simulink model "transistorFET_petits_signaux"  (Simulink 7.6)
settings: Solver=ode15s  StartTime=0.0  StopTime=0.06  RelTol=1e-3
InitFcn:
  | clc
  | RD=1000;
libraries: fl_lib x7, nesl_utility x3, AppliElectrical_lib x1

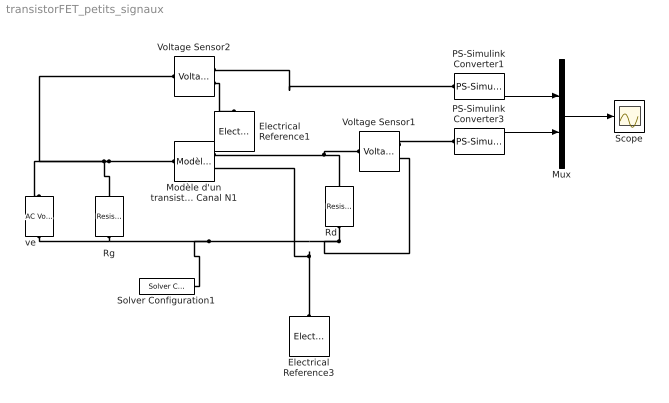
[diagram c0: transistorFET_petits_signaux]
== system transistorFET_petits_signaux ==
  Electrical Reference1 : fl_lib/Electrical/Electrical Elements/Electrical Reference  DialogController=NetworkEngine.DynNeDlgSource  SystemSampleTime=-1  i_Log=off  LocalVarNames=|i  LocalVarDescs=|i  LocalVarLogging=0
  Electrical Reference3 : fl_lib/Electrical/Electrical Elements/Electrical Reference  DialogController=NetworkEngine.DynNeDlgSource  SystemSampleTime=-1  i_Log=off  LocalVarNames=|i  LocalVarDescs=|i  LocalVarLogging=0
  Modèle d'un transistor à effet de champ Canal N1 : AppliElectrical_lib/Modèle d'un transistor à effet de champ Canal N  DialogController=NetworkEngine.DynNeDlgSource  SystemSampleTime=-1  g=0.003 A/V  rho=1e+6 Ohm  ie_Log=off  vgs_Log=off  is_Log=off  vds_Log=off  LocalVarNames=|ie|vgs|is|vds  LocalVarDescs=|courant d'entrée du FET|tension, Grille-Source|courant Drain-Source|tension Drain-Source  LocalVarLogging=[0 0 0 0]
  Mux : Mux  Inputs=2
  PS-Simulink Converter1 : nesl_utility/PS-Simulink Converter  DialogController=NetworkEngine.DynNeUtilDlgSource  SystemSampleTime=-1  PhysicalDomain=network_engine_domain  LeftPortType=input  RightPortType=output  SubClassName=ps_output  Unit=1  AffineConversion=off
  PS-Simulink Converter3 : nesl_utility/PS-Simulink Converter  DialogController=NetworkEngine.DynNeUtilDlgSource  SystemSampleTime=-1  PhysicalDomain=network_engine_domain  LeftPortType=input  RightPortType=output  SubClassName=ps_output  Unit=1  AffineConversion=off
  Rd : fl_lib/Electrical/Electrical Elements/Resistor  DialogController=NetworkEngine.DynNeDlgSource  SystemSampleTime=-1  R=1 kOhm  i_Log=off  v_Log=off  LocalVarNames=|i|v  LocalVarDescs=|i|v  LocalVarLogging=[0 0]
  Rg : fl_lib/Electrical/Electrical Elements/Resistor  DialogController=NetworkEngine.DynNeDlgSource  SystemSampleTime=-1  R=1 MOhm  i_Log=off  v_Log=off  LocalVarNames=|i|v  LocalVarDescs=|i|v  LocalVarLogging=[0 0]
  Scope : Scope
  Solver Configuration1 : nesl_utility/Solver Configuration  DialogController=NetworkEngine.DynNeUtilDlgSource  SystemSampleTime=-1  PhysicalDomain=network_engine_domain  LeftPortType=input  RightPortType=generic  SubClassName=solver  Accelerate=off  Profile=off  ResidualTolerance=1e-9  MaxNonlinIter=3  MaxModeIter=2  DoFixedCost=off  UseLocalSampling=off  DoDC=off  LinearAlgebra=Sparse  LocalSolverSampleTime=.001  LocalSolverChoice=NE_BACKWARD_EULER_ADVANCER  UseLocalSolver=off
  Voltage Sensor1 : fl_lib/Electrical/Electrical Sensors/Voltage Sensor  DialogController=NetworkEngine.DynNeDlgSource  SystemSampleTime=-1  i1_Log=off  v1_Log=off  LocalVarNames=|i1|v1  LocalVarDescs=|i1|v1  LocalVarLogging=[0 0]
  Voltage Sensor2 : fl_lib/Electrical/Electrical Sensors/Voltage Sensor  DialogController=NetworkEngine.DynNeDlgSource  SystemSampleTime=-1  i1_Log=off  v1_Log=off  LocalVarNames=|i1|v1  LocalVarDescs=|i1|v1  LocalVarLogging=[0 0]
  ve : fl_lib/Electrical/Electrical Sources/AC Voltage Source  DialogController=NetworkEngine.DynNeDlgSource  SystemSampleTime=-1  amp=10 mV  shift=0 rad  omega=60 Hz  i_Log=off  v_Log=off  LocalVarNames=|i|v  LocalVarDescs=|i|v  LocalVarLogging=[0 0]
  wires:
  PS-Simulink Converter3/1 -> Mux/2
  Mux/1 -> Scope/1
  PS-Simulink Converter1/1 -> Mux/1
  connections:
  Voltage Sensor1/RConn1 -- PS-Simulink Converter3/LConn1
  Voltage Sensor2/RConn2 -- Electrical Reference1/LConn1
  Modèle d'un transistor à effet de champ Canal N1/LConn1 -- ve/LConn1 -- Voltage Sensor2/LConn1 -- Rg/RConn1
  Voltage Sensor2/RConn1 -- PS-Simulink Converter1/LConn1
  Modèle d'un transistor à effet de champ Canal N1/RConn1 -- Voltage Sensor1/LConn1 -- Rd/RConn1
  ve/RConn1 -- Modèle d'un transistor à effet de champ Canal N1/RConn2 -- Electrical Reference3/LConn1 -- Rd/LConn1 -- Voltage Sensor1/RConn2 -- Solver Configuration1/RConn1 -- Rg/LConn1
